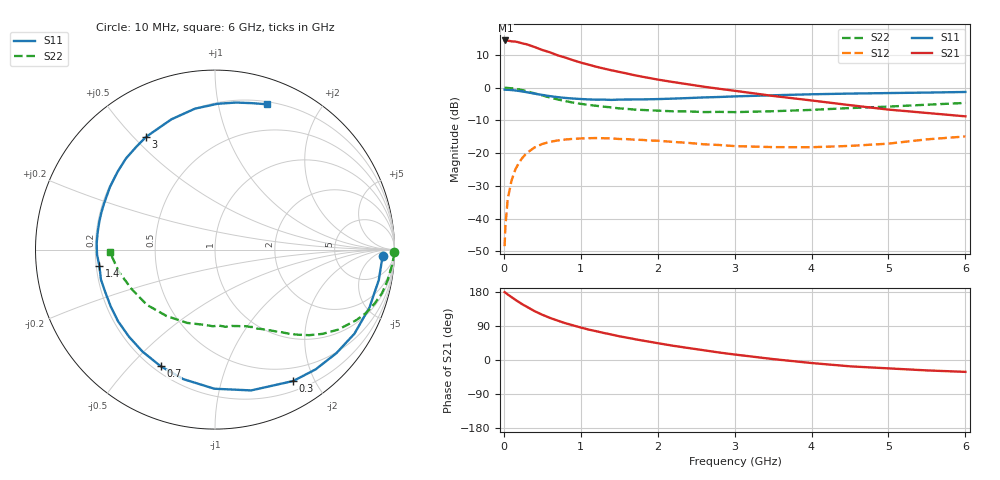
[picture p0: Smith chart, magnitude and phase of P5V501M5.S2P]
! SIEMENS Small Signal Semiconductors
! BFP183
! Si NPN RF Bipolar Junction Transistor in SOT143
! VCE = 0.5 V  IC = 1.5 mA
! Common Emitter S-Parameters:  March  1996
# GHz  S  MA  R  50
!  f  S11  S21  S12  S22
! GHz  MAG  ANG  MAG  ANG  MAG  ANG  MAG  ANG
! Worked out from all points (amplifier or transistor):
!   36 points, 10 MHz to 6 GHz, reference 50 ohm
!   highest |S21| = 14.4 dB at 20 MHz (marker M1)
!   |S21| within 3 dB of that: start of sweep to 512.7 MHz
!   unconditionally stable (mu >= 1): 2.075 GHz to end of sweep
!   at 250 MHz: K = 0.13, MSG = 17.3 dB, |S12| = -21.2 dB
!   at 1.4 GHz: K = 0.67, MSG = 10.4 dB, |S12| = -15.5 dB
!   at 6 GHz: K = 1.29, MAG = -0.2 dB, |S12| = -14.9 dB
!   S11 on the Smith chart (normalised r, x): 10 MHz: 23, -13; 300 MHz: 0.32, -1.72; 700 MHz: 0.23, -0.61; 1.4 GHz: 0.21, -0.07; 3 GHz: 0.20, +0.54; 6 GHz: 0.22, +1.40
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0.01  0.9353 -2.1  5.19 179.0  0.0038 85.5  0.9974 -0.9
0.02  0.9308 -4.4  5.262 177.8  0.0076 82.7  0.9974 -2.0
0.05  0.9282 -10.5  5.231 172.9  0.0197 84.2  0.9904 -4.9
0.1  0.919 -20.5  5.103 166.0  0.0383 77.2  0.9778 -9.7
0.15  0.9072 -31.1  5.058 158.9  0.0565 71.4  0.9623 -14.5
0.2  0.8889 -40.5  4.906 152.3  0.0727 66.2  0.9388 -18.7
0.3  0.8521 -59.2  4.59 140.3  0.1009 55.8  0.8803 -26.5
0.4  0.81 -75.6  4.176 128.9  0.1222 46.6  0.8185 -33.0
0.5  0.7751 -90.3  3.765 119.4  0.1381 39.1  0.7611 -38.1
0.6  0.7429 -103.8  3.463 111.1  0.1491 32.7  0.7084 -42.3
0.7  0.7168 -115.0  3.119 103.9  0.1564 27.3  0.6614 -45.8
0.8  0.6972 -125.4  2.881 97.1  0.1616 22.5  0.6236 -48.7
0.9  0.6822 -134.6  2.63 91.4  0.1653 18.6  0.5915 -51.1
1.1  0.6618 -151.4  2.251 80.4  0.1692 11.8  0.5453 -55.6
1.4  0.6505 -171.8  1.843 67.1  0.1679 3.6  0.5 -61.8
1.7  0.6608 171.6  1.549 55.1  0.1606 -1.3  0.4629 -67.4
2.2  0.6811 149.3  1.219 37.6  0.1486 -6.6  0.4358 -77.5
3  0.7361 121.5  0.897 14.5  0.1282 -7.5  0.4233 -97.4
3.5  0.7654 108.5  0.748 2.4  0.1237 -3.9  0.4369 -110.8
4.5  0.8125 89.0  0.541 -16.7  0.1291 5.0  0.4885 -140.9
5.5  0.8416 75.8  0.411 -27.5  0.1625 9.5  0.5498 -167.0
6  0.8599 70.3  0.365 -31.3  0.1799 7.5  0.585 -178.5
